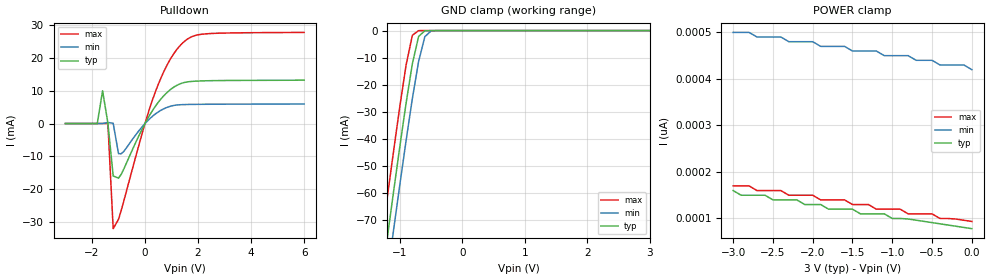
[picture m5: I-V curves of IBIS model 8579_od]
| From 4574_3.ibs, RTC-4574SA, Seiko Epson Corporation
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|   Model 8579_od
[Model]   8579_od
Model_type   Open_drain
Polarity   Inverting
C_comp   8.00pF   8.00pF   8.00pF
[Temperature Range]   25.00   85.00   -40.00
[Voltage Range]   3.00V   2.70V   3.30V
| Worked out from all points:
|   slope of the pulldown table from 0 to 0.45 V, typ, clamps not added: 75.9 ohm
|   GND clamp passes 1 mA (typ) near -0.64 V on its own axis
[Pulldown]
| voltage   I(typ)   I(min)   I(max)
-3V       0A         0A         0A
-1.8V     0A         0A         0A
-1.6V     10mA       0A         0A
-1.4V     140uA      320uA      0A
-1.2V     -16.02mA   70uA       -32.1mA
-1V       -16.67mA   -9.18mA    -29.25mA
-900mV    -15.55mA   -9.24mA    -26.63mA
400mV     5.37mA     2.97mA     9.86mA
900mV     9.97mA     5.13mA     18.87mA
1.4V      12.34mA    5.76mA     24.44mA
2.2V      13.03mA    5.87mA     27.31mA
6V        13.24mA    5.96mA     27.82mA
[GND_clamp]
| voltage   I(typ)   I(min)   I(max)
-3V       -400mA     -410mA     -380mA
-1.3V     -93.61mA   -110mA     -78.67mA
-1.2V     -76.37mA   -90.58mA   -61.4mA
-1.1V     -59.37mA   -73.57mA   -44.4mA
-1V       -42.73mA   -56.83mA   -27.91mA
-900mV    -26.73mA   -40.55mA   -12.63mA
-800mV    -12.21mA   -25.06mA   -1.72mA
-700mV    -2.15mA    -11.34mA   -18.92uA
-600mV    -68.39uA   -2.24mA    -130nA
-500mV    -1.41uA    -130uA     -900pA
3V        3pA        15.06pA    3pA
[POWER_clamp]
| voltage   I(typ)   I(min)   I(max)
-3V       160pA      500pA      170pA
-2.9V     150pA      500pA      170pA
-2.6V     150pA      490pA      160pA
-2.5V     140pA      490pA      160pA
-2.2V     140pA      480pA      150pA
-2.1V     130pA      480pA      150pA
-1.6V     120pA      470pA      140pA
-1.1V     110pA      450pA      120pA
-900mV    100pA      450pA      120pA
-800mV    98.95pA    450pA      110pA
-700mV    96.35pA    440pA      110pA
0V        78.15pA    420pA      93.6pA
[Ramp]
| variable   typ   min   max
dV/dt_r   1.57/4.88n   1.11/9.08n   2.00/2.95n
dV/dt_f   1.57/4.88n   1.11/9.08n   2.00/2.95n
R_load = 0.50k
| End [Model] 8579_od
| End [Component] RTC-4574SA
